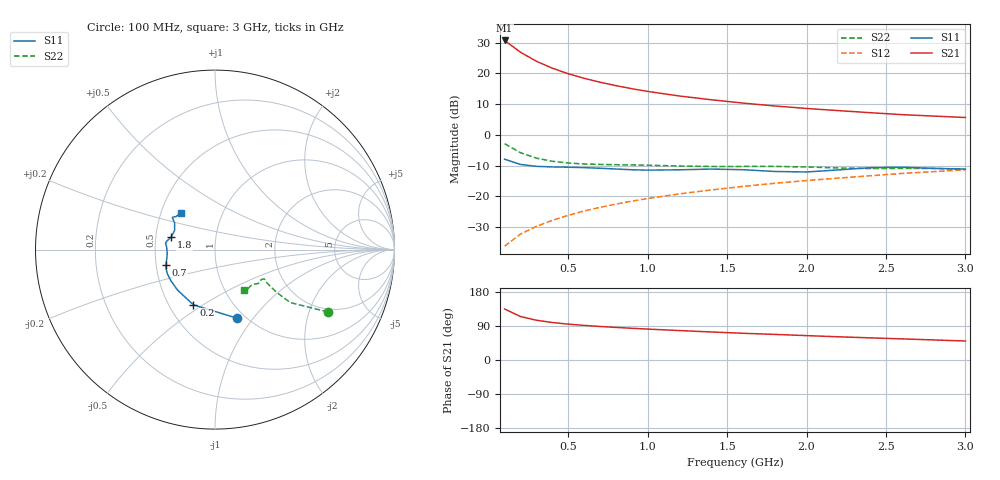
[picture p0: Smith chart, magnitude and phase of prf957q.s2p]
! Filename:  PRF957Q.S2P  Version:  3.0
! Philips part #:  PRF957  Date:  Nov 1998
! Bias condition:  Vce=6V, Ic=30mA
#  MHz  S  MA  R 50
! Freq  S11  S21  S12  S22
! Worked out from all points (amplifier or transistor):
!   20 points, 100 MHz to 3 GHz, reference 50 ohm
!   highest |S21| = 30.7 dB at 100 MHz (marker M1)
!   |S21| within 3 dB of that: start of sweep to 178.3 MHz
!   unconditionally stable (mu >= 1): 675.2 MHz to end of sweep
!   at 400 MHz: K = 0.93, MSG = 24.7 dB, |S12| = -27.8 dB
!   at 1.2 GHz: K = 1.04, MAG = 14.6 dB, |S12| = -19.2 dB
!   at 3 GHz: K = 1.03, MAG = 7.5 dB, |S12| = -11.4 dB
!   lowest NFmin = 1.85 dB at 500 MHz
!   S11 on the Smith chart (normalised r, x): 100 MHz: 0.92, -0.84; 200 MHz: 0.66, -0.46; 700 MHz: 0.56, -0.11; 1.8 GHz: 0.60, +0.09; 3 GHz: 0.64, +0.28
100  0.4018 -72.1  34.14 134.6  0.01552 69.2  0.7185 -28.9
200  0.3303 -111.4  21.97 114.7  0.02442 67.9  0.5122 -35.1
300  0.3074 -132.6  15.68 105.0  0.03251 70.3  0.4182 -34.8
400  0.301 -145.0  12.11 98.9  0.04079 72.4  0.3719 -33.6
500  0.2978 -152.8  9.842 94.7  0.0492 74.1  0.3482 -32.8
600  0.2933 -158.1  8.292 91.3  0.05774 75.2  0.336 -32.3
700  0.2864 -162.4  7.163 88.5  0.0663 76.0  0.3302 -31.9
800  0.2783 -166.6  6.304 86.0  0.07492 76.5  0.3271 -31.5
900  0.2708 -171.0  5.62 83.7  0.08353 77.0  0.3241 -31.1
1000  0.2668 -175.6  5.078 81.6  0.09228 77.1  0.3207 -30.9
1200  0.2702 176.7  4.272 77.7  0.1098 77.1  0.3117 -31.6
1400  0.2777 172.4  3.716 74.0  0.1271 76.8  0.3057 -34.0
1600  0.271 169.6  3.28 70.5  0.145 76.4  0.3062 -36.5
1800  0.2539 164.1  2.943 67.6  0.1633 75.7  0.3067 -38.0
2000  0.249 154.6  2.681 64.4  0.1807 75.1  0.3006 -39.2
2200  0.2691 146.6  2.475 61.2  0.1979 74.4  0.2895 -41.8
2400  0.2923 143.7  2.289 58.4  0.2161 73.5  0.283 -45.8
2600  0.2978 142.8  2.129 55.8  0.2359 72.4  0.2844 -49.5
2800  0.2848 139.8  2.016 52.9  0.2523 71.8  0.2843 -51.6
3000  0.2777 132.3  1.912 50.0  0.2701 71.1  0.2764 -53.5
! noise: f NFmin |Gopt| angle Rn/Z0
500  1.85  0.08  -161  0.26
800  2.19  0.23  171  0.08
900  2.22  0.26  163  0.1
1000  2.28  0.18  141  0.2
1500  2.2  0.39  143  0.15
2000  2.57  0.34  -139  0.23
